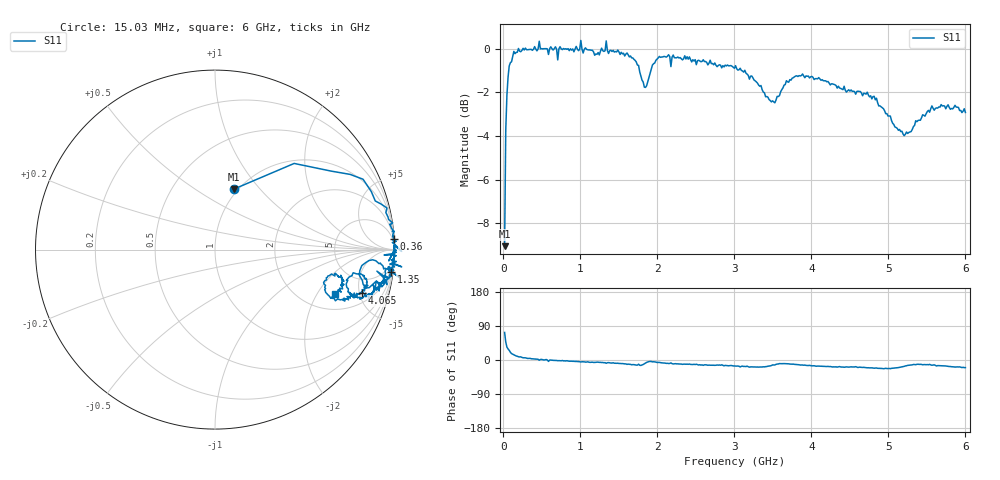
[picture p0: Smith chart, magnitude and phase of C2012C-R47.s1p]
!	Network	Analyzer	HP8753E.07.74:	Oct	30	2002	Serial	No.	JP38451487
!	Hewlett-Packard
!	28	Aug	2009	12:02:15
!	Frequency	S11
#	HZ	S	RI	R	50
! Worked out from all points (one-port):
!   400 points, 15.03 MHz to 6 GHz, reference 50 ohm
!   lowest |S11| = -9.0 dB at 15.03 MHz (marker M1), VSWR 2.09, Z = 47.9 + j36.8 ohm
!   |S11| at or under -10 dB: nowhere
!   S11 on the Smith chart (normalised r, x): 15.03 MHz: 0.96, +0.74; 360 MHz: 2, +33; 1.35 GHz: 1, -16; 4.065 GHz: 2.96, -5.30; 6 GHz: 2.90, -2.92
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1.502992e7  0.105 0.337
3.002985e7  0.441 0.48
4.502978e7  0.649 0.437
9.002955e7  0.871 0.323
1.95029e8  0.99 0.149
3.600282e8  0.995 0.0593
5.550272e8  1 0.0225
5.850271e8  0.968 -0.0627
6.00027e8  1 -0.00403
7.050265e8  0.942 -0.03
7.650262e8  0.995 -0.0233
1.350023e9  0.983 -0.124
1.515022e9  0.958 -0.153
1.725021e9  0.907 -0.217
1.830021e9  0.804 -0.143
1.90502e9  0.878 -0.0568
2.02502e9  0.954 -0.107
2.265019e9  0.942 -0.169
3.015015e9  0.878 -0.255
3.315013e9  0.781 -0.266
3.480013e9  0.731 -0.191
3.765011e9  0.843 -0.161
4.06501e9  0.819 -0.242
4.515007e9  0.765 -0.249
4.935005e9  0.671 -0.285
5.265004e9  0.624 -0.155
5.565002e9  0.718 -0.177
6e9  0.671 -0.246
